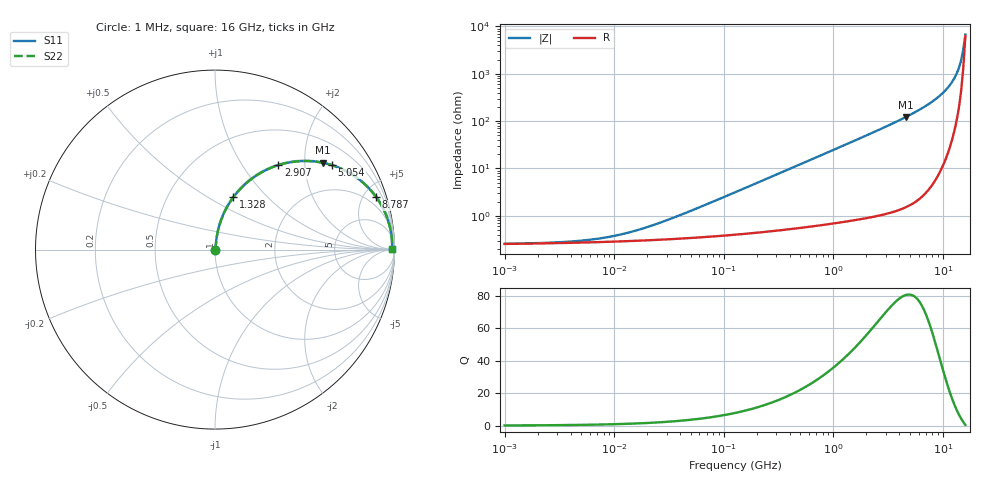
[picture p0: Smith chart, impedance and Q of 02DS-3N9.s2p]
# MHz S MA R 50
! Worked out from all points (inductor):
!   211 points, 1 MHz to 16 GHz, reference 50 ohm
!   read as one part in series: L = 3.9 nH near 41.84 MHz
!   highest Q = 80.7 at 4.609 GHz (marker M1), where L = 4.24 nH
!   S11 on the Smith chart (normalised r, x): 1 MHz: 1.01, +0.00; 1.328 GHz: 1.02, +0.66; 2.907 GHz: 1.02, +1.47; 5.054 GHz: 1.03, +2.75; 8.787 GHz: 1.13, +6.11; 16 GHz: open
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1  0.002545 5.5  0.9975 -0.0  0.9975 -0.0  0.002545 5.5
5.25662  0.003002 25.3  0.9973 -0.1  0.9973 -0.1  0.003002 25.3
11.5091  0.004016 44.3  0.9971 -0.2  0.9971 -0.2  0.004016 44.3
26.3872  0.007157 63.9  0.9969 -0.4  0.9969 -0.4  0.007157 63.9
132.458  0.03256 81.1  0.9955 -1.9  0.9955 -1.9  0.03256 81.1
333.021  0.08112 81.9  0.9918 -4.6  0.9918 -4.6  0.08112 81.9
664.915  0.1602 78.7  0.9812 -9.2  0.9812 -9.2  0.1602 78.7
1327.58  0.3092 70.7  0.9439 -18.0  0.9439 -18.0  0.3092 70.7
2010.19  0.4443 62.6  0.888 -26.4  0.888 -26.4  0.4443 62.6
2906.66  0.5888 53.1  0.7998 -36.1  0.7998 -36.1  0.5888 53.1
3187.38  0.6265 50.4  0.7708 -38.8  0.7708 -38.8  0.6265 50.4
4608.83  0.7711 38.8  0.6272 -50.4  0.6272 -50.4  0.7711 38.8
5053.93  0.8035 35.8  0.5854 -53.5  0.5854 -53.5  0.8035 35.8
6978.58  0.8979 25.3  0.4273 -63.9  0.4273 -63.9  0.8979 25.3
8787.49  0.9446 18.0  0.3091 -70.8  0.3091 -70.8  0.9446 18.0
11065.3  0.9737 11.0  0.1911 -76.6  0.1911 -76.6  0.9737 11.0
12134  0.9808 8.3  0.1445 -78.2  0.1445 -78.2  0.9808 8.3
13305.8  0.9852 5.6  0.09823 -78.5  0.09823 -78.5  0.9852 5.6
13933.5  0.9865 4.3  0.07536 -77.5  0.07536 -77.5  0.9865 4.3
14590.9  0.9871 3.0  0.05282 -74.4  0.05282 -74.4  0.9871 3.0
15279.2  0.9871 1.6  0.03115 -64.8  0.03115 -64.8  0.9871 1.6
16000  0.9866 0.3  0.01457 -22.5  0.01457 -22.5  0.9866 0.3
